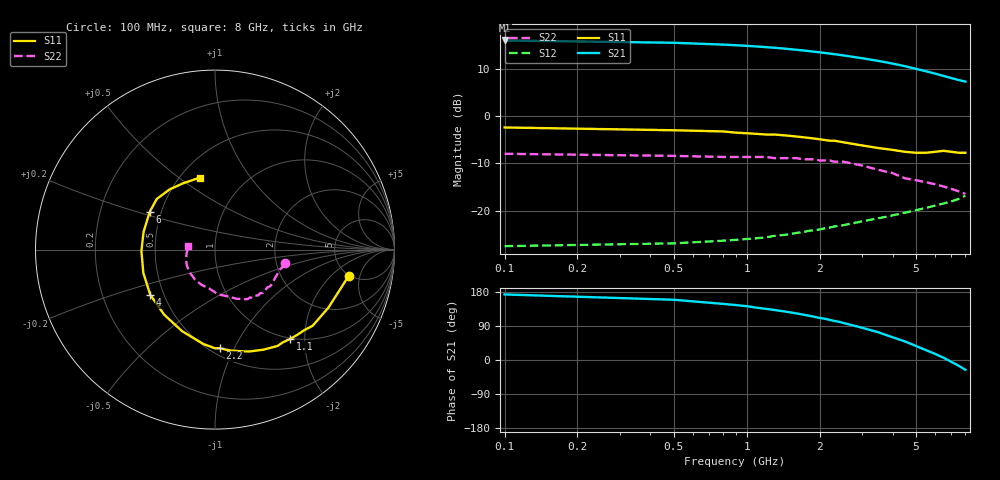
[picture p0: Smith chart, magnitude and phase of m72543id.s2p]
!  MGA-72543 S PARAMETERS
!  Vd=3V  Id=20 mA Vc=0.5V  LAST UPDATED 01-27-99
# ghz s ma r 50
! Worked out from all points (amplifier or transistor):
!   31 points, 100 MHz to 8 GHz, reference 50 ohm
!   highest |S21| = 16.1 dB at 100 MHz (marker M1)
!   |S21| within 3 dB of that: start of sweep to 2.373 GHz
!   unconditionally stable (mu >= 1): start of sweep to end of sweep
!   at 1.1 GHz: K = 1.16, MAG = 17.9 dB, |S12| = -25.8 dB
!   at 2.1 GHz: K = 1.17, MAG = 16.1 dB, |S12| = -23.7 dB
!   at 8 GHz: K = 1.33, MAG = 8.6 dB, |S12| = -16.8 dB
!   lowest NFmin = 1.30 dB at 800 MHz
!   S11 on the Smith chart (normalised r, x): 100 MHz: 4.94, -3.39; 1.1 GHz: 0.98, -1.70; 2.2 GHz: 0.56, -0.88; 4 GHz: 0.42, -0.26; 6 GHz: 0.43, +0.22; 8 GHz: 0.62, +0.60
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0.1  0.76 -11.0  6.35 173.0  0.042 18.0  0.4 -11.0
0.5  0.71 -27.0  6.001 159.0  0.045 12.0  0.38 -17.0
0.8  0.69 -38.0  5.738 148.0  0.048 15.0  0.37 -25.0
0.9  0.67 -42.0  5.65 145.0  0.049 16.0  0.37 -27.0
1  0.66 -46.0  5.569 142.0  0.05 17.0  0.37 -29.0
1.1  0.65 -50.0  5.481 138.0  0.051 18.0  0.37 -32.0
1.4  0.63 -60.0  5.231 129.0  0.055 19.0  0.36 -38.0
1.6  0.61 -67.0  5.064 123.0  0.058 19.0  0.36 -42.0
1.9  0.58 -77.0  4.826 114.0  0.062 20.0  0.35 -47.0
2.2  0.55 -87.0  4.613 106.0  0.066 19.0  0.34 -52.0
2.5  0.53 -97.0  4.412 98.0  0.07 18.0  0.33 -57.0
3  0.49 -112.0  4.112 85.0  0.077 16.0  0.3 -66.0
3.5  0.46 -128.0  3.851 73.0  0.083 13.0  0.27 -75.0
4  0.44 -145.0  3.613 60.0  0.089 10.0  0.25 -86.0
4.5  0.42 -162.0  3.391 49.0  0.095 6.0  0.22 -98.0
5  0.41 -179.0  3.179 37.0  0.101 2.0  0.21 -111.0
5.5  0.41 166.0  2.995 26.0  0.107 -1.0  0.2 -124.0
6  0.42 150.0  2.825 16.0  0.113 -5.0  0.19 -138.0
6.5  0.43 139.0  2.672 6.0  0.119 -10.0  0.18 -151.0
7  0.42 127.0  2.534 -5.0  0.125 -14.0  0.17 -162.0
7.5  0.41 116.0  2.42 -15.0  0.133 -18.0  0.16 -172.0
8  0.41 102.0  2.329 -26.0  0.144 -23.0  0.15 172.0
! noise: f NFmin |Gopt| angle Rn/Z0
0.8  1.3  0.37  39  0.25
1  1.32  0.35  41  0.22
1.8  1.38  0.22  58  0.2
2  1.39  0.21  65  0.19
2.2  1.41  0.2  71  0.19
2.4  1.43  0.2  78  0.18
3  1.45  0.18  95  0.17
4  1.47  0.16  139  0.14
5  1.54  0.18  -175  0.12
6  1.67  0.27  -129  0.14
